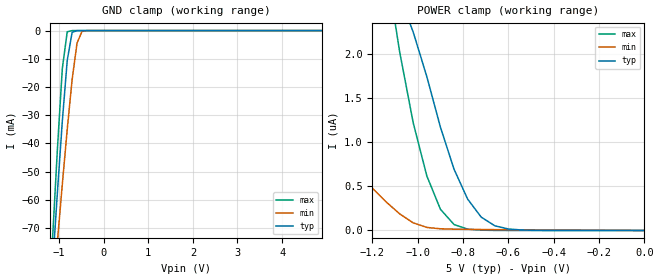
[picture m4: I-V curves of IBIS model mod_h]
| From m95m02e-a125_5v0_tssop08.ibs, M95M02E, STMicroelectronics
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|   Model mod_h
[Model]   mod_h
Model_type Input
Vinl   =   1.500V
Vinh   =   3.500V
C_comp   3.207pF   3.063pF   3.358pF
[Temperature Range]  25.0000   0.1250k   -40.0000
[Voltage Range]   5.0000V   4.5000V   5.5000V
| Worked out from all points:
|   GND clamp passes 1 mA (typ) near -0.71 V on its own axis
[GND_clamp]
|Voltage   I(typ)   I(min)   I(max)
-5V       -1.086A    -869.4mA   -1.312A
-1.15V    -83.9mA    -95.65mA   -74.15mA
-1.04V    -57.37mA   -74.82mA   -41.97mA
-930mV    -32.19mA   -54.5mA    -13.5mA
-820mV    -10.62mA   -35.06mA   -423.4uA
-710mV    -641.8uA   -17.42mA   -3.991uA
-600mV    -10.98uA   -4.462mA   -43.85nA
-490mV    -174.9nA   -327.6uA   -197pA
-270mV    -39.85pA   -578.3nA   -4.242pA
4.9V      78.49pA    5.426nA    77.56pA
[POWER_clamp]
|Voltage   I(typ)   I(min)   I(max)
-4.98V    11.16uA    6.056uA    19.16uA
-1.86V    6.388uA    2.345uA    12.89uA
-1.8V     6.147uA    2.181uA    12.52uA
-1.14V    3.021uA    324.9nA    3.013uA
-1.08V    2.658uA    188.7nA    2.027uA
-1.02V    2.25uA     86.43nA    1.22uA
-960mV    1.745uA    34.43nA    618.2nA
-900mV    1.172uA    19.12nA    240.7nA
-840mV    695.1nA    14.85nA    67.41nA
-720mV    151.4nA    11.06nA    3.483nA
-600mV    16.65nA    8.455nA    251.8pA
0V        80.2pA     516.7pA    87.5pA
